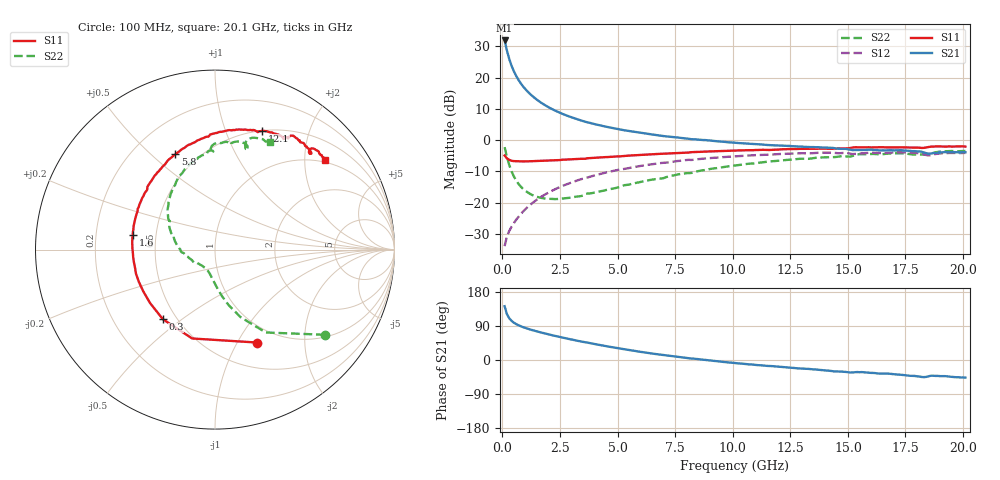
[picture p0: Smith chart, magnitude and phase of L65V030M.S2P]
!  Infineon Technologies AG
! BFR380L3 , PF131585-7, No.6, Th 09.10.01, soldered on pcb-board, measured with PP GSG850
!  Vce=5.0 V,  Ic=30.0 mA
! Common Emitter S-Parameters:  15. November 2001
#  GHz  S  MA  R  50
! f  S11  S21  S12  S22
! GHz  Mag  Ang  Mag  Ang  Mag  Ang  Mag  Ang
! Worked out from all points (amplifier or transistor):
!   201 points, 100 MHz to 20.1 GHz, reference 50 ohm
!   highest |S21| = 31.9 dB at 100 MHz (marker M1)
!   |S21| within 3 dB of that: start of sweep to 193.6 MHz
!   unconditionally stable (mu >= 1): 1.26 GHz to 4.344 GHz
!   at 3.4 GHz: K = 1.02, MAG = 8.6 dB, |S12| = -12.5 dB
!   at 10.1 GHz: K = 0.95, MSG = 2.2 dB, |S12| = -5.2 dB
!   at 20.1 GHz: K = 0.99, MSG = 0.1 dB, |S12| = -4.1 dB
!   S11 on the Smith chart (normalised r, x): 100 MHz: 0.79, -1.21; 300 MHz: 0.42, -0.43; 1.6 GHz: 0.37, +0.08; 5.8 GHz: 0.38, +0.60; 12.1 GHz: 0.50, +1.35; 20.1 GHz: 0.95, +2.50
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0.1  0.5683 -65.7  39.18 141.9  0.02023 63.6  0.7739 -37.8
0.2  0.5112 -104.4  27.08 121.1  0.02898 56.8  0.5415 -58.5
0.3  0.4846 -126.8  19.87 110.2  0.03532 56.5  0.4018 -69.3
0.4  0.4686 -140.5  15.5 103.4  0.04138 57.6  0.3178 -76.3
0.5  0.4624 -150.0  12.65 98.5  0.04706 59.6  0.2643 -81.2
0.6  0.4607 -157.2  10.66 94.9  0.05338 61.2  0.2276 -85.1
0.7  0.4602 -163.0  9.209 91.7  0.05935 62.5  0.2008 -88.5
0.8  0.4568 -167.5  8.108 89.1  0.06583 63.8  0.1814 -91.5
0.9  0.4573 -171.4  7.235 86.7  0.07228 64.4  0.1663 -94.1
1.1  0.458 -177.8  5.971 82.6  0.08547 65.4  0.1463 -99.4
1.3  0.4615 176.9  5.083 78.9  0.0986 65.8  0.1328 -104.1
1.6  0.4651 170.1  4.164 73.8  0.1186 65.6  0.1217 -111.0
2  0.4733 162.2  3.37 67.8  0.145 64.5  0.1155 -119.7
2.4  0.4805 155.2  2.843 62.1  0.1717 62.9  0.1148 -128.3
3.5  0.5032 139.1  2.018 47.9  0.2429 56.7  0.1303 -147.7
5.8  0.575 112.6  1.345 23.4  0.3762 41.8  0.2076 175.2
6.8  0.6029 103.0  1.19 14.5  0.4275 34.6  0.243 162.0
10.1  0.6827 78.7  0.9088 -8.1  0.5513 13.1  0.3936 129.1
12.1  0.7131 68.3  0.8181 -18.2  0.6016 1.0  0.4726 111.6
13.5  0.7315 61.2  0.7757 -24.7  0.6219 -7.7  0.5148 101.1
16.8  0.7667 48.5  0.6904 -36.2  0.6309 -23.9  0.6108 79.5
20.1  0.7887 39.1  0.6404 -46.4  0.6258 -37.8  0.6715 62.9
